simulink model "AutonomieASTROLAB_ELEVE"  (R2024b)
settings: Solver=VariableStepAuto  StartTime=0.0  StopTime=86400  RelTol=1e-3  AbsTol=1e-3  EnableMultiTasking=on
libraries: fl_lib x15, batteryecm_lib x8, nesl_utility x3

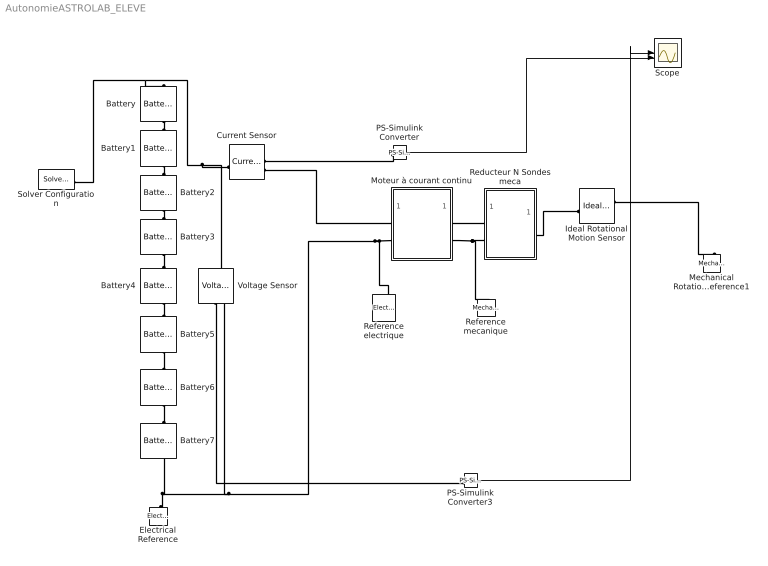
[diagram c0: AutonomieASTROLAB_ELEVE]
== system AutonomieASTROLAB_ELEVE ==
  Battery{,1..7} (8 alike) : batteryecm_lib/Battery  Vnom=2 V  prm_dir=simscape.enum.battery.prm_dir.disabled  R1_dis=2 Ohm  R1_ch=2 Ohm  R1=0.1 Ohm  prm_AH=simscape.enum.battery.prm_AH.finite  AH=0.5 A*hr  V1=1.4 V  AH1=0.1 A*hr  prm_R2=simscape.enum.battery.prm_R2.disabled  R2=2000 Ohm  Tmeas=298.15 K  charge_measurement_port=simscape.enum.battery.enable.no  prm_dyn=simscape.enum.battery.prm_dyn.off  Rp1=0.005 Ohm  tau1=30 s  Rp2=0.005 Ohm  tau2=30 s  Rp3=0.005 Ohm  tau3=30 s  Rp4=0.005 Ohm  tau4=30 s  Rp5=0.005 Ohm  tau5=30 s  prm_fade=simscape.enum.battery.prm_fade.disabled  N_fade=100  AH_fade=45 A*hr  R1_fade=2.02 Ohm  R1_ch_fade=2.02 Ohm  V1_fade=10.35 V  prm_age=simscape.enum.battery.prm_age.disabled  prm_age_OCV=simscape.enum.battery.prm_age_OCV.OCV  OCV_age=0.9  SOC_age=60  Tmeas_age=298.15 K  delta_time_age_vec=[0] d  temperature_age_vec=[273] K  OCV_scaling_age=2.2134e6  OCV_offset_age=1.632e6  temp_exp_age=0.515833569 V  t_exp_age=0.75  Vnom_T2=12 V  R1_T2=2.2 Ohm  R1_T2_dis=2.2 Ohm  R1_T2_ch=2.2 Ohm  V1_T2=11.4 V  R2_T2=2200 Ohm  Rp1_T2=0.005 Ohm  tau1_T2=30 s  Rp2_T2=0.005 Ohm  tau2_T2=30 s  Rp3_T2=0.005 Ohm  tau3_T2=30 s  Rp4_T2=0.005 Ohm  tau4_T2=30 s  Rp5_T2=0.005 Ohm  tau5_T2=30 s  Tmeas2=273.15 K  thermal_port=simscape.enum.thermaleffects.omit  thermal_mass=30000 J/K  i_specify=off  i_priority=None  i=0 A  i_nominal_specify=off  i_nominal_value=1  i_nominal_unit=A  v_specify=off  v_priority=None  v=0 V  v_nominal_specify=off  v_nominal_value=1  v_nominal_unit=V  charge_specify=on  charge_priority=High  charge=2.6 A*hr  charge_nominal_specify=off  charge_nominal_value=2.6  charge_nominal_unit=A*hr  num_cycles_specify=off  num_cycles_priority=High  num_cycles=0  num_cycles_nominal_specify=off  num_cycles_nominal_value=1  num_cycles_nominal_unit=1  temperature_specify=off  temperature_priority=High  temperature=298.15 K  temperature_nominal_specify=off  temperature_nominal_value=1  temperature_nominal_unit=K
  Current Sensor : fl_lib/Electrical/Electrical Sensors/Current Sensor
  Electrical Reference : fl_lib/Electrical/Electrical Elements/Electrical Reference
  Ideal Rotational Motion Sensor : fl_lib/Mechanical/Mechanical Sensors/Ideal Rotational Motion Sensor  reference=foundation.enum.MeasurementReference.difference  acceleration_port=false  velocity_port=true  position_port=true  wrap_angle=false  offset=0 rad
  Mechanical Rotational Reference1 : fl_lib/Mechanical/Rotational Elements/Mechanical Rotational Reference
  Moteur à courant continu : Subsystem
  PS-Simulink Converter : nesl_utility/PS-Simulink Converter  PhysicalDomain=network_engine_domain  SubClassName=ps_output  LeftPortType=input  RightPortType=output  PseudoPeriodic=off  Frequencies=[]  VectorFormat=inherit  Unit=A  AffineConversion=off
  PS-Simulink Converter3 : nesl_utility/PS-Simulink Converter  PhysicalDomain=network_engine_domain  SubClassName=ps_output  LeftPortType=input  RightPortType=output  PseudoPeriodic=off  Frequencies=[]  VectorFormat=inherit  Unit=V  AffineConversion=off
  Reducteur N Sondes meca : Subsystem
  Reference electrique : fl_lib/Electrical/Electrical Elements/Electrical Reference
  Reference mecanique : fl_lib/Mechanical/Rotational Elements/Mechanical Rotational Reference
  Scope : Scope  NumInputPorts=2
  Solver Configuration : nesl_utility/Solver Configuration  PhysicalDomain=network_engine_domain  SubClassName=solver  LeftPortType=input  RightPortType=generic  Tones=[]  Harmonics=[]  SimulateNoise=off  Profile=off  UseLocalSampling=off  EnableSwitchedLinearOptims=on  FrequencyDomain=off  UseCCode=off  RelTol=0.001  AbsTol=1e-06  MinStep=1e-09  ToWorkspace=off  RevertToSquareIcSolve=off  NumHomotopyIterations=100  PhasorMode=off  PhasorModeNumHarmonics=1  ConsistencySolver=NEWTON_XTOL_AFTER_FTOL  IndexReductionMethod=DerivativeReplacement  DoDC=off  ResidualTolerance=1e-09  ConsistencyTolSource=GLOBAL  ConsistencyAbsTol=0.001  ConsistencyRelTol=0.001  ConsistencyTolFactor=0.001  UseLocalSolver=off  LocalSolverChoice=NE_BACKWARD_EULER_ADVANCER  ResolveIndetEquations=on  FunctionEvalNumThread=1  LocalSolverSampleTime=0.001  DoFixedCost=off  MaxNonlinIter=3  MaxModeIter=2  ComputeImpulses=off  ImpulseIterations=2  LinearAlgebra=auto  LinearAlgebraNumThread=0  EquationFormulation=NE_TIME_EF  DelaysMemoryBudget=1024  AutomaticFiltering=on  FilteringTimeConstant=0.001  PartitionStorageMethod=AS_NEEDED  PartitionMemoryBudget=1024  PartitionMethod=ROBUST  MultibodyUseLocalSolver=off  MultibodyLocalSolverChoice=ODE1  MultibodyLocalSolverSampleTime=0.001
  Voltage Sensor : fl_lib/Electrical/Electrical Sensors/Voltage Sensor
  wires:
  PS-Simulink Converter3/1 -> Scope/1
  PS-Simulink Converter/1 -> Scope/2
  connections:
  Solver Configuration/RConn1 -- Voltage Sensor/LConn1 -- Current Sensor/LConn1 -- Battery/LConn1
  Battery2/LConn1 -- Battery1/RConn1
  Battery1/LConn1 -- Battery/RConn1
  Battery5/LConn1 -- Battery4/RConn1
  Battery3/RConn1 -- Battery4/LConn1
  Moteur à courant continu/LConn2 -- Battery7/RConn1 -- Electrical Reference/LConn1 -- Voltage Sensor/RConn2 -- Reference electrique/LConn1
  PS-Simulink Converter/LConn1 -- Current Sensor/RConn1
  Battery5/RConn1 -- Battery6/LConn1
  Battery6/RConn1 -- Battery7/LConn1
  Ideal Rotational Motion Sensor/RConn1 -- Mechanical Rotational Reference1/LConn1
  Voltage Sensor/RConn1 -- PS-Simulink Converter3/LConn1
  Battery3/LConn1 -- Battery2/RConn1
  Reducteur N Sondes meca/LConn2 -- Reference mecanique/LConn1 -- Moteur à courant continu/RConn2
  Current Sensor/RConn2 -- Moteur à courant continu/LConn1
  Moteur à courant continu/RConn1 -- Reducteur N Sondes meca/LConn1
  Reducteur N Sondes meca/RConn1 -- Ideal Rotational Motion Sensor/LConn1

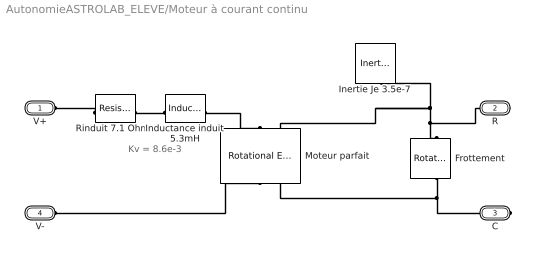
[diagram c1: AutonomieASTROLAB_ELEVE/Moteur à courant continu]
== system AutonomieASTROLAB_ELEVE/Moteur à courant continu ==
  note: Kv = 8.6e-3
  Frottement : fl_lib/Mechanical/Rotational Elements/Rotational Friction  brkwy_trq=5.7e-4 N*m  brkwy_vel=0.030296 rad/s  Col_trq=2.7e-4 N*m  visc_coef=1.7e-7 N*m/(rad/s)  w_specify=off  w_priority=None  w=0 rad/s  w_nominal_specify=off  w_nominal_value=1  w_nominal_unit=rad/s  t_specify=off  t_priority=None  t=0 N*m  t_nominal_specify=off  t_nominal_value=1  t_nominal_unit=N*m
  Inductance induit 5.3mH : fl_lib/Electrical/Electrical Elements/Inductor  l=5.3 mH  r=0 Ohm  g=1e-09 1/Ohm  i_specify=off  i_priority=None  i=0 A  i_nominal_specify=off  i_nominal_value=1  i_nominal_unit=A  v_specify=off  v_priority=None  v=0 V  v_nominal_specify=off  v_nominal_value=1  v_nominal_unit=V  i_L_specify=on  i_L_priority=High  i_L=0 A  i_L_nominal_specify=off  i_L_nominal_value=1  i_L_nominal_unit=A
  Inertie Je 3.5e-7 : fl_lib/Mechanical/Rotational Elements/Inertia  inertia=3.5 g*cm^2  num_ports=foundation.enum.numPorts2.one  w_specify=on  w_priority=High  w=0 rad/s  w_nominal_specify=off  w_nominal_value=1  w_nominal_unit=rad/s  t_specify=off  t_priority=None  t=0 N*m  t_nominal_specify=off  t_nominal_value=1  t_nominal_unit=N*m
  Moteur parfait : fl_lib/Electrical/Electrical Elements/Rotational Electromechanical Converter  K=8.6e-3 V/(rad/s)  i_specify=off  i_priority=None  i=0 A  i_nominal_specify=off  i_nominal_value=1  i_nominal_unit=A  v_specify=off  v_priority=None  v=0 V  v_nominal_specify=off  v_nominal_value=1  v_nominal_unit=V  t_specify=off  t_priority=None  t=0 N*m  t_nominal_specify=off  t_nominal_value=1  t_nominal_unit=N*m  w_specify=off  w_priority=None  w=0 rad/s  w_nominal_specify=off  w_nominal_value=1  w_nominal_unit=rad/s
  Rinduit 7.1 Ohms : fl_lib/Electrical/Electrical Elements/Resistor  Tag=Factory Generic  R=7.1 Ohm  i_specify=off  i_priority=None  i=0 A  i_nominal_specify=off  i_nominal_value=1  i_nominal_unit=A  v_specify=off  v_priority=None  v=0 V  v_nominal_specify=off  v_nominal_value=1  v_nominal_unit=V
  V+ : PMIOPort  Side=Left
  R : PMIOPort  Port=2  Side=Right
  C : PMIOPort  Port=3  Side=Right
  V- : PMIOPort  Port=4  Side=Left
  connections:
  Moteur parfait/LConn1 -- Inductance induit 5.3mH/RConn1
  V-/RConn1 -- Moteur parfait/RConn1
  Rinduit 7.1 Ohms/LConn1 -- V+/RConn1
  Inductance induit 5.3mH/LConn1 -- Rinduit 7.1 Ohms/RConn1
  Frottement/LConn1 -- Moteur parfait/LConn2 -- Inertie Je 3.5e-7/LConn1 -- R/RConn1
  Frottement/RConn1 -- Moteur parfait/RConn2 -- C/RConn1

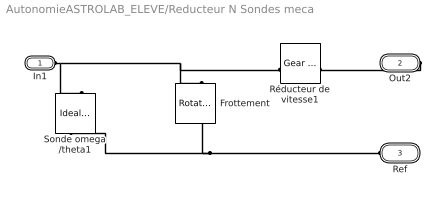
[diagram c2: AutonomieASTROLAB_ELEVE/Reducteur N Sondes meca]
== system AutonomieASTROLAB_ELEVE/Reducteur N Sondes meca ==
  Frottement : fl_lib/Mechanical/Rotational Elements/Rotational Friction  brkwy_trq=1e-3 N*m  brkwy_vel=0.030296 rad/s  Col_trq=0.35e-3 N*m  visc_coef=1.7e-7 N*m/(rad/s)  w_specify=off  w_priority=None  w=0 rad/s  w_nominal_specify=off  w_nominal_value=1  w_nominal_unit=rad/s  t_specify=off  t_priority=None  t=0 N*m  t_nominal_specify=off  t_nominal_value=1  t_nominal_unit=N*m
  Réducteur de vitesse1 : fl_lib/Mechanical/Mechanisms/Gear Box  ratio=12320  t_in_specify=off  t_in_priority=None  t_in=0 N*m  t_in_nominal_specify=off  t_in_nominal_value=1  t_in_nominal_unit=N*m  t_out_specify=off  t_out_priority=None  t_out=0 N*m  t_out_nominal_specify=off  t_out_nominal_value=1  t_out_nominal_unit=N*m
  Sonde omega /theta1 : fl_lib/Mechanical/Mechanical Sensors/Ideal Rotational Motion Sensor  reference=foundation.enum.MeasurementReference.difference  acceleration_port=false  velocity_port=true  position_port=true  wrap_angle=false  offset=0 rad
  In1 : PMIOPort  Side=Left
  Out2 : PMIOPort  Port=2  Side=Right
  Ref : PMIOPort  Port=3  Side=Left
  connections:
  Out2/RConn1 -- Réducteur de vitesse1/RConn1
  Ref/RConn1 -- Sonde omega /theta1/RConn1 -- Frottement/RConn1
  In1/RConn1 -- Sonde omega /theta1/LConn1 -- Réducteur de vitesse1/LConn1 -- Frottement/LConn1
